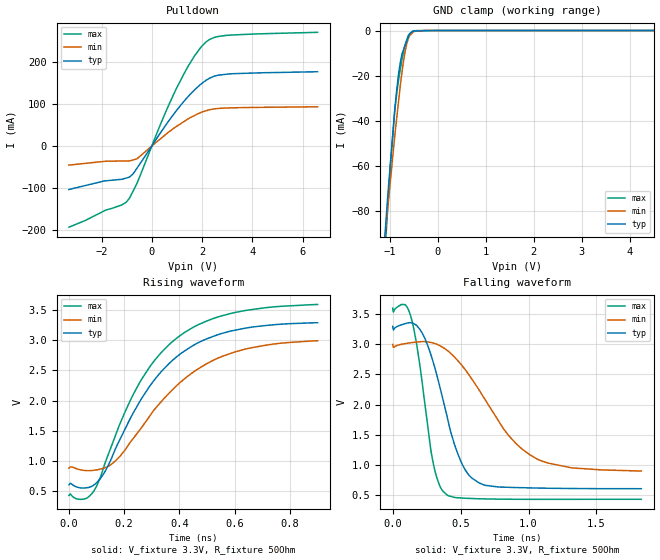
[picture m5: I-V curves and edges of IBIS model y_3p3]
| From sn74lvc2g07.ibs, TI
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|   y_3p3 Model
[Model]   y_3p3
Model_type   Open_drain
Polarity   Non-Inverting
Vmeas = 1.65
Vref = 3.3
Cref = 2pF
Rref = 1200
|   typ   min   max
|   (nom PVT)   (fast PVT)   (slow PVT)
|C_comp from frequency sweep method (F=5MHz)
C_comp   4.932e-12   4.666e-12   4.948e-12
|ON state : BUFFER OUTPUT TURNED LOW
|C_comp   4.932e-12   4.666e-12   4.948e-12
|OFF state: BUFFER IN HIGH IMPEDANCE
|C_comp   3.354e-12   3.341e-12   3.359e-12
|C_comp from LC tank measurement(L=1nH)
|Resonant Frequency(Hz)   2.690e+09   2.730e+09   2.520e+09
|C_comp   3.504e-12   3.402e-12   3.993e-12
|ON state : BUFFER OUTPUT TURNED LOW
|Resonant Frequency(Hz)   2.690e+09   2.730e+09   2.520e+09
|C_comp   3.504e-12   3.402e-12   3.993e-12
|OFF state: BUFFER IN HIGH IMPEDANCE
|Resonant Frequency(Hz)   2.770e+09   2.780e+09   2.770e+09
|C_comp   3.305e-12   3.281e-12   3.305e-12
| Where nom  PVT is Nominal Process, 3.3V, 27C
|   Fast PVT is Strong Process,  3.6V, -40C
|   Slow PVT is Weak Process,   3V, 125C
[Voltage Range]   3.3   3   3.6
|Ambient Temperature   25   85   -40
|Junction Temperature
[Temperature Range]   27   125   -40
[Pullup Reference]   3.3   3   3.6
[Pulldown Reference]   0   0   0
[Power Clamp Reference]   3.3   3   3.6
[GND Clamp Reference]   0   0   0
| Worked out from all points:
|   slope of the pulldown table from 0 to 0.495 V, typ, clamps not added: 11.2 ohm
|   GND clamp passes 1 mA (typ) near -0.56 V on its own axis
|   falling waveform, V_fixture 3.3V, R_fixture 50Ohm: 20-80 % time 196ps typ, 391ps min, 117ps max; typ from 3.3 V to 0.604 V
|   rising waveform, V_fixture 3.3V, R_fixture 50Ohm: 20-80 % time 235ps typ, 262ps min, 232ps max; typ from 0.605 V to 3.29 V
[Pulldown]
|   Voltage   I(typ)   I(min)   I(max)
-3.3V     -103.8mA   -45.63mA   -193.4mA
-1.884V   -83.29mA   -36.67mA   -154.3mA
-1.206V   -79.54mA   -35.96mA   -140.8mA
-896.4mV  -74.41mA   -35.78mA   -125.2mA
-591mV    -52.87mA   -30.53mA   -89.02mA
331.2mV   30.19mA    16.4mA     49.52mA
939.6mV   81.03mA    44.73mA    131.8mA
1.703V    133.6mA    72.57mA    214.6mA
2.167V    156.7mA    83.9mA     248mA
2.473V    165.9mA    88.17mA    258.2mA
2.934V    170.5mA    90.29mA    263.1mA
6.6V      176.8mA    93.27mA    270.6mA
[GND Clamp]
|   Voltage   I(typ)   I(min)   I(max)
-3.3V     -864mA     -702mA     -1.025A
-1.141V   -102.5mA   -101.6mA   -112.1mA
-1.071V   -81.48mA   -84.82mA   -87.8mA
-993.6mV  -60.29mA   -67.8mA    -61.01mA
-896.4mV  -34.88mA   -46.45mA   -35.19mA
-856.8mV  -26.31mA   -38.8mA    -27.93mA
-785.4mV  -14.55mA   -25.02mA   -17.53mA
-745.8mV  -10.29mA   -18.3mA    -12.68mA
-681mV    -6.593mA   -9.161mA   -6.242mA
-606mV    -2.318mA   -3.017mA   -1.991mA
-525.6mV  -475.6uA   -953uA     -231.9uA
6.6V      0A         0A         0A
[POWER Clamp]
|   Voltage   I(typ)   I(min)   I(max)
-3.3V     0A         0A         0A
0V        0A         0A         0A
6.6V      0A         0A         0A
[Ramp]
R_load = 1200
|   typ   min   max
dV/dt_r   1.96241/5.48308e-09   1.77162/5.49176e-09   2.14828/5.4587e-09
dV/dt_f   1.96248/1.57664e-10   1.77168/2.91083e-10   2.14835/1.0116e-10
[Falling Waveform]
V_fixture = 3.3V
V_fixture_min = 3V
V_fixture_max = 3.6V
R_fixture = 50Ohm
|   Time   V(typ)   V(min)   V(max)
0s        3.3V       3V         3.6V
130ps     3.36V      3.026V     3.488V
185ps     3.292V     3.04V      2.874V
295ps     2.727V     3.024V     1.064V
395ps     1.852V     2.91V      508.9mV
530ps     930.6mV    2.591V     445.1mV
675ps     663mV      2.101V     434.5mV
860ps     626.2mV    1.47V      428.5mV
1.07ns    614.3mV    1.089V     427.2mV
1.83ns    603.8mV    897mV      428.2mV
[Rising Waveform]
V_fixture = 3.3V
V_fixture_min = 3V
V_fixture_max = 3.6V
R_fixture = 50Ohm
|   Time   V(typ)   V(min)   V(max)
0s        605.1mV    880.6mV    428.2mV
55ps      551.2mV    842.5mV    368.5mV
90ps      599.9mV    844.3mV    500.6mV
160ps     1.108V     967.6mV    1.32V
235ps     1.814V     1.387V     2.122V
310ps     2.348V     1.855V     2.667V
390ps     2.727V     2.249V     3.035V
495ps     3.018V     2.602V     3.312V
600ps     3.166V     2.805V     3.46V
900ps     3.291V     2.992V     3.593V
